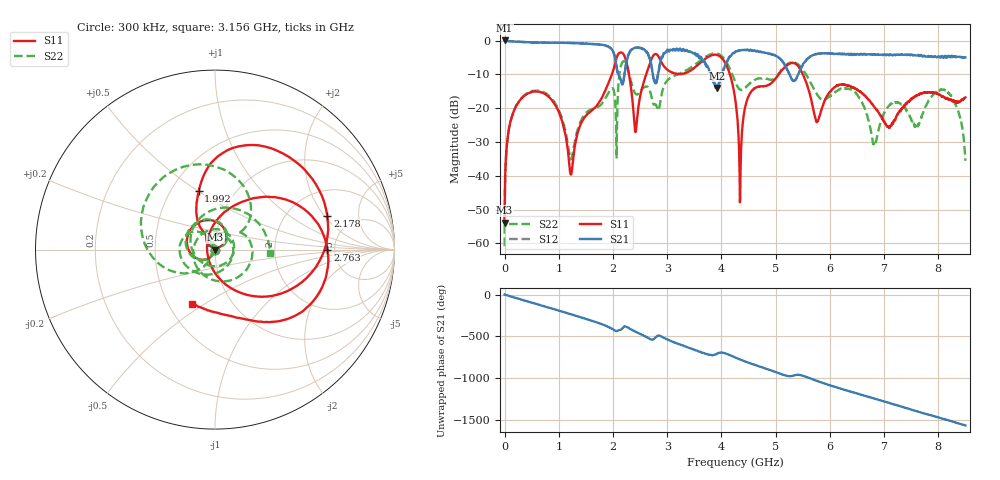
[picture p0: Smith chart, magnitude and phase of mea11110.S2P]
!Agilent Technologies,E5071B,MY42402595,A.08.01
!Date: Tue Jan 02 09:24:05 2001
!Data & Calibration Information:
!Freq	S11:SOLT2(ON)	S21:SOLT2(ON)	S12:SOLT2(ON)	S22:SOLT2(ON)
# Hz S dB R 50
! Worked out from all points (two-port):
!   1601 points, 300 kHz to 8.5 GHz, reference 50 ohm
!   highest |S21| = 0.08 dB at 300 kHz (marker M1); lowest = -14.0 dB at 3.915 GHz (marker M2)
!   |S21| within 3 dB of the highest: start of sweep to 1.993 GHz; 2.328 GHz to 2.591 GHz (262.9 MHz wide, 10.7 % of centre)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
!   lowest |S11| = -53.8 dB at 300 kHz (marker M3), VSWR 1.00, Z = 50.2 - j0.0329 ohm
!   |S11| at or under -10 dB: start of sweep to 1.978 GHz; 4.157 GHz to 5.054 GHz (897.3 MHz wide, 19.5 % of centre); 5.501 GHz to end of sweep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
!   |S22| runs from -60.8 to -3.7 dB; largest |S21 - S12| = 0.052
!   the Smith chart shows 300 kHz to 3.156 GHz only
!   S11 on the Smith chart (normalised r, x): 300 kHz: 1.00, -0.00; 1.992 GHz: 0.68, +0.51; 2.178 GHz: 3.26, +2.15; 2.763 GHz: 4.36, -0.02; 3.156 GHz: 0.66, -0.44
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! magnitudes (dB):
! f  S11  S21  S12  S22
! 300 kHz  -53.8  0.1  0.0  -60.8
! 79.98 MHz  -26.1  -0.1  -0.1  -26.1
! 308.4 MHz  -17.2  -0.3  -0.4  -17.0
! 903.4 MHz  -18.3  -0.6  -0.6  -17.8
! 1.222 GHz  -39.6  -0.7  -0.7  -35.1
! 1.419 GHz  -24.2  -0.8  -0.8  -23.3
! 1.992 GHz  -9.4  -2.9  -3.0  -14.1
! 2.178 GHz  -3.7  -12.9  -13.0  -6.2
! 2.417 GHz  -27.0  -2.1  -2.0  -15.7
! 2.763 GHz  -4.1  -12.1  -11.5  -18.9
! 2.837 GHz  -4.6  -9.4  -9.3  -20.6
! 3.156 GHz  -9.7  -2.7  -2.8  -10.2
! 3.915 GHz  -4.2  -14.0  -13.2  -3.8
! 4.25 GHz  -16.9  -3.4  -3.4  -12.0
! 4.346 GHz  -46.8  -2.8  -2.8  -14.5
! 4.521 GHz  -15.7  -2.9  -2.8  -12.7
! 5.228 GHz  -7.1  -9.0  -8.9  -6.8
! 5.669 GHz  -18.2  -4.4  -4.4  -13.1
! 6.821 GHz  -19.6  -4.1  -4.0  -30.9
! 7.087 GHz  -25.7  -4.3  -4.2  -19.3
! 8.139 GHz  -16.9  -4.7  -4.9  -14.8
! 8.5 GHz  -16.8  -5.0  -5.0  -35.6
